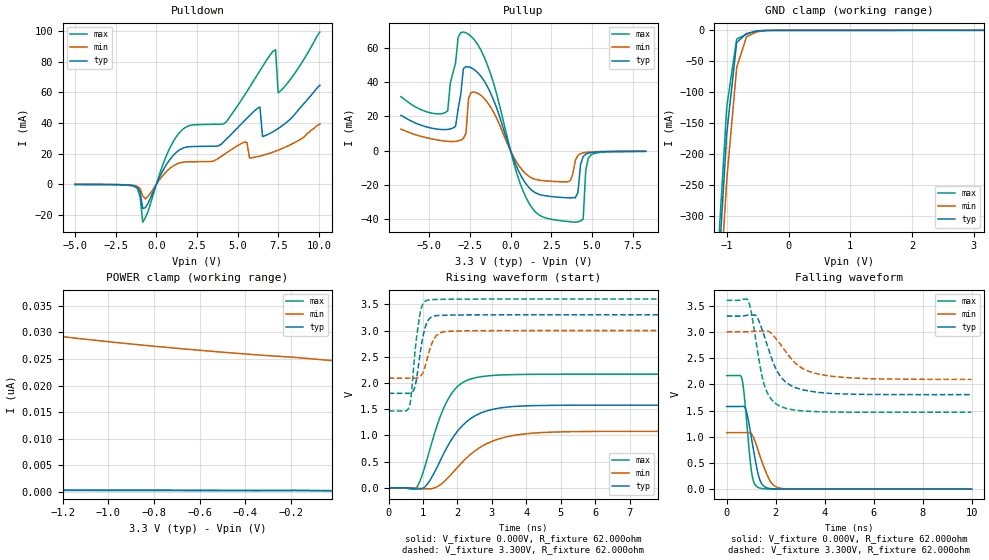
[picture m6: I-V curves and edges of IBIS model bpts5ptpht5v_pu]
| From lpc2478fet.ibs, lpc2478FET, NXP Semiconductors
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| bpts5ptpht5v
|   Bidirectional Pad 3v3
|   CMOS
|   Characterized at Core 1.8V and I/O 3.3V
| Pull Up Mode (p1=0, p2=0)
[Model]   bpts5ptpht5v_pu | of bpts5ptpht5v
Model_type   I/O
Polarity   Non-Inverting
Enable   Active-Low
|  Reciever Thresholds
Vinl   = 0.54V
Vinh   = 1.26V
| AC Test Load Conditions
Vref   = 0
Cref   = 1.2e-11
Rref   = 1000000000
Vmeas   = 0.9
| [Process Range]   typical   min   max
| C_comp edge width   400.000ps   400.000ps   400.000ps
| C_comp Tstrobe   40.000fs   40.000fs   40.000fs
C_comp   2.521pF   2.387pF   2.657pF
[Temperature Range]   25   125   -40
[Voltage Range]   3.30V   3.00V   3.60V
[GND Clamp Reference]   0.00V   0.00V   0.00V
[Pulldown Reference]   0.00V   0.00V   0.00V
[POWER Clamp Reference]   3.30V   3.00V   3.60V
[Pullup Reference]   3.30V   3.00V   3.60V
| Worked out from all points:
|   slope of the pulldown table from 0 to 0.495 V, typ, clamps not added: 46.5 ohm
|   slope of the pullup table from 0 to 0.495 V, typ, clamps not added: 41.9 ohm
|   GND clamp passes 1 mA (typ) near -0.48 V on its own axis
|   rising waveform, V_fixture 0.000V, R_fixture 62.000ohm: 20-80 % time 918ps typ, 1.16ns min, 699ps max; typ from 0.001 V to 1.58 V
|   falling waveform, V_fixture 0.000V, R_fixture 62.000ohm: 20-80 % time 365ps typ, 510ps min, 257ps max; typ from 1.58 V to 0.001 V
|   rising waveform, V_fixture 3.300V, R_fixture 62.000ohm: 20-80 % time 221ps typ, 261ps min, 201ps max; typ from 1.8 V to 3.3 V
|   falling waveform, V_fixture 3.300V, R_fixture 62.000ohm: 20-80 % time 805ps typ, 1.12ns min, 531ps max; typ from 3.3 V to 1.8 V
[GND Clamp]
| ref voltage   0.00V   0.00V   0.00V
|   Voltage   I(typ)   I(min)   I(max)
-5V       -7.933A    -7.953A    -7.929A
-1.16V    -429.6mA   -501mA     -389.4mA
-1V       -166mA     -240.8mA   -123.1mA
-840mV    -19.71mA   -60.08mA   -14.11mA
-680mV    -5.176mA   -10.17mA   -6.124mA
-520mV    -1.303mA   -2.648mA   -850.4uA
-200mV    -54.41uA   -43.67uA   -84.58uA
3.16V     195.7pA    25.28nA    129.9pA
[Power Clamp]   | Vtable = Vcc - Vpad
| ref voltage   3.30V   3.00V   3.60V
|   Voltage   I(typ)   I(min)   I(max)
-6.74V    1.25nA     124.2nA    594.5pA
-4.66V    764.3pA    69.65nA    461.2pA
-2.42V    442.5pA    37.56nA    320.3pA
-2.26V    425.1pA    36.17nA    310.3pA
-2.1V     408.2pA    34.87nA    300.3pA
-1.78V    376pA      32.56nA    280.3pA
-1.46V    345.7pA    30.59nA    260.3pA
-1.14V    316.9pA    28.91nA    240.4pA
-660mV    276.2pA    26.86nA    210.5pA
-340mV    250.5pA    25.75nA    190.5pA
-180mV    238.9pA    25.3nA     243pA
-20mV     211pA      24.7nA     154.4pA
[Pulldown]
| ref voltage   0.00V   0.00V   0.00V
|   Voltage   I(typ)   I(min)   I(max)
-5V       -187.5uA   -145.7uA   -211.8uA
-1.32V    -1.32mA    -939.4uA   -1.723mA
-1V       -5.322mA   -2.96mA    -8.616mA
-840mV    -15.95mA   -7.733mA   -24.9mA
1.4V      22.26mA    13.79mA    33.48mA
4.28V     29.27mA    20.27mA    40.55mA
5.56V     43.15mA    27.33mA    60.63mA
6.36V     50.49mA    18.36mA    74.24mA
6.52V     31.16mA    18.79mA    76.97mA
7.32V     35.27mA    21.55mA    87.95mA
7.48V     36.36mA    22.22mA    59.78mA
10.04V    64.68mA    39.32mA    99.49mA
[Pullup]   | Vtable = Vcc - Vpad
| ref voltage   3.30V   3.00V   3.60V
|   Voltage   I(typ)   I(min)   I(max)
-6.74V    20.65mA    12.57mA    31.52mA
-3.86V    12.45mA    5.473mA    23.29mA
-3.22V    24.39mA    5.73mA     66.13mA
-2.9V     47.88mA    7.139mA    69.22mA
-2.42V    48.4mA     34.05mA    66.69mA
780mV     -16.88mA   -11.92mA   -23.75mA
2.38V     -26.56mA   -17.72mA   -39.7mA
3.98V     -27.38mA   -5.509mA   -41.66mA
4.46V     -3.36mA    -1.235mA   -39.9mA
4.62V     -2.02mA    -961.4uA   -11.27mA
4.94V     -1.105mA   -662.3uA   -2.417mA
8.3V      -310.5uA   -276uA     -365.2uA
[Ramp]
R_load   = 62.000ohm
|   dV/dt(typ)   dV/dt(min)   dV/dt(max)
dV/dt_r   723.911mV/915.000ps   486.077mV/1.125ns   1.052V/765.000ps
dV/dt_f   678.844mV/810.000ps   404.699mV/1.100ns   1.039V/585.000ps
[Rising Waveform]  | cubic spline decimation from 2001 points
V_fixture   = 0.000V
R_fixture   = 62.000ohm
|   Time   V(typ)   V(min)   V(max)
0s        1.319mV    1.084mV    1.611mV
820ps     -19.3mV    -4.63mV    17.02mV
1.13ns    76.64mV    -18.33mV   576mV
1.445ns   447.1mV    36.02mV    1.261V
1.685ns   760.3mV    165.4mV    1.639V
1.99ns    1.073V     384.6mV    1.926V
2.375ns   1.318V     636.9mV    2.074V
3.03ns    1.499V     894.6mV    2.144V
4.05ns    1.565V     1.036V     2.164V
10ns      1.577V     1.079V     2.167V
[Falling Waveform]  | cubic spline decimation from 2001 points
V_fixture   = 0.000V
R_fixture   = 62.000ohm
|   Time   V(typ)   V(min)   V(max)
0s        1.577V     1.079V     2.167V
620ps     1.579V     1.079V     2.11V
805ps     1.485V     1.08V      1.346V
1.015ns   967.4mV    1.051V     329.7mV
1.115ns   695.2mV    965.2mV    127.8mV
1.29ns    279.7mV    730.7mV    32.36mV
1.48ns    74.96mV    474.4mV    11.17mV
1.775ns   13.37mV    156.1mV    4.603mV
2.235ns   3.864mV    16.8mV     2.815mV
10ns      1.32mV     1.09mV     1.611mV
[Rising Waveform]  | cubic spline decimation from 2001 points
V_fixture   = 3.300V
V_fixture_min = 3.000V
V_fixture_max = 3.600V
R_fixture   = 62.000ohm
|   Time   V(typ)   V(min)   V(max)
0s        1.803V     2.092V     1.467V
595ps     1.803V     2.093V     1.54V
650ps     1.812V     2.092V     1.728V
755ps     1.907V     2.092V     2.517V
890ps     2.443V     2.114V     3.234V
975ps     2.81V      2.171V     3.477V
1.1ns     3.131V     2.414V     3.573V
1.36ns    3.281V     2.881V     3.592V
1.715ns   3.293V     2.984V     3.597V
10ns      3.3V       3V         3.6V
[Falling Waveform]  | cubic spline decimation from 2001 points
V_fixture   = 3.300V
V_fixture_min = 3.000V
V_fixture_max = 3.600V
R_fixture   = 62.000ohm
|   Time   V(typ)   V(min)   V(max)
0s        3.3V       3V         3.6V
880ps     3.318V     3.001V     3.59V
995ps     3.32V      3.006V     3.396V
1.19ns    3.309V     3.014V     2.842V
1.53ns    2.926V     3.014V     1.997V
1.805ns   2.536V     2.979V     1.727V
2.155ns   2.177V     2.786V     1.588V
3ns       1.909V     2.33V      1.497V
3.825ns   1.842V     2.187V     1.476V
10ns      1.803V     2.093V     1.467V
